(* Logix 5000 AddOnInstructionDefinition export Bronkhorst_FF_Extended_INT_Input; software revision 37.00 *)

ADD_ON_INSTRUCTION Bronkhorst_FF_Extended_INT_Input   (* revision 1.0, vendor Bronkhorst High-Tech B.V. *)
// Extract data from the FLEXI-FLOW Extended INT input connection (in to controller from device)
VAR_IN_OUT
   DataIn : SINT[16]; {required}
END_VAR
VAR_OUTPUT
   Status : USINT; {visible}
   Measure : INT; {visible}
   Setpoint : INT; {visible}
   Override : USINT; {visible}
   Actuator : UINT; {visible}
   Pressure_Inlet : INT; {visible}
   Pressure_Inlet_Setpoint : INT; {visible}
   Pressure_Outlet : INT; {visible}
   Pressure_Outlet_Setpoint : INT; {visible}
END_VAR

ROUTINE Logic   (* structured text *)
   Status := DataIn[0];
   COP(DataIn[1], Measure, 1);
   COP(DataIn[3], Setpoint, 1);
   Override := DataIn[5];
   COP(DataIn[6], Actuator , 1);
   COP(DataIn[8], Pressure_Inlet, 1);
   COP(DataIn[10], Pressure_Inlet_Setpoint, 1);
   COP(DataIn[12], Pressure_Outlet, 1);
   COP(DataIn[14], Pressure_Outlet_Setpoint, 1);
END_ROUTINE
END_ADD_ON_INSTRUCTION

ADD_ON_INSTRUCTION Bronkhorst_FF_Extended_INT_Output   (* revision 1.0, vendor Bronkhorst High-Tech B.V. *)
// Fill data for the FLEXI-FLOW Extended INT output connection (out from controller to device)
VAR_IN_OUT
   DataOut : SINT[7]; {required}
END_VAR
VAR_INPUT
   Override : USINT; {visible}
   Setpoint : INT; {visible}
   Pressure_Inlet_Setpoint : INT; {visible}
   Pressure_Outlet_Setpoint : INT; {visible}
END_VAR

ROUTINE Logic   (* structured text *)
   DataOut[0] := Override;
   COP(Setpoint, DataOut[1], 2);
   COP(Pressure_Inlet_Setpoint, DataOut[3], 2);
   COP(Pressure_Outlet_Setpoint, DataOut[5], 2);
END_ROUTINE
END_ADD_ON_INSTRUCTION
